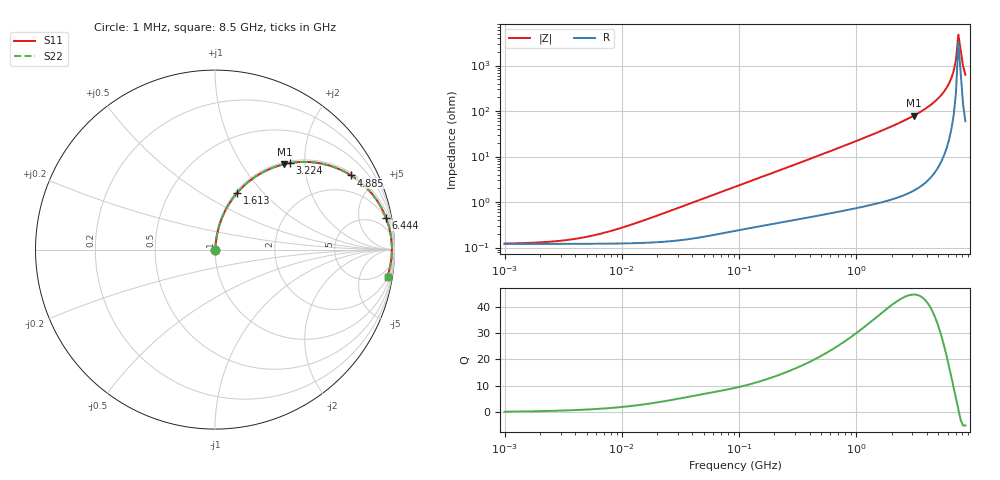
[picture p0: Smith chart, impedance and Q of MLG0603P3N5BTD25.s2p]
! S-Parameter Data Generated by TDK Corporation
! Copyright(C) 2025 TDK Corporation.
! All Rights Reserved.
! TDK P/N: MLG0603P3N5BTD25 (SMD / SMT Inductor (Coil))
! Property: L=3.5nH at 500MHz
! Size(LxWxT): 0.6x0.3x0.3mm
! Model Type: s2p (Touchstone File Format Version 1.0)
! Frequency: DC=Yes Start=1MHz Stop=8500MHz 198points Log-sweep
! Model Generated on Feb. 6, 2025
! Terms and conditions regarding TDK Simulation Models:
! 1)This simulation model is being provided solely for informational
!  purposes. Please refer to the specifications of the products in
!  terms of detailed characteristics of such products.
! 2)In no event shall TDK Corporation of any of its subsidiaries be
!  liable for any loss or damage arising, directly or indirectly,
!  from any information contained in this simulation model, including,
!  but not limited to loss or damages arising from any inaccuracies,
!  omissions or errors in connection with such information.
! 3)Any and all copyrights on this simulation model are owned by
!  TDK Corporation.  Duplication or redistribution of this simulation
!  model without prior written permission from TDK Corporation
!  is prohibited.
! 4)This simulation model is subject to any modification or change
!  without any prior notice.
! 5)Neither TDK Corporation nor any of its subsidiaries shall make any
!  warranty, express or implied, including but not limited to the
!  correctness, implied warranties of merchantability and fitness for
!  a particular purpose with respect to this simulation models.
! 6)The use of this simulation model shall be deemed to have consented
!  to the terms and conditions hereof.
! Port Assignments:
!  1 ---@@@--- 2
! Applicable Conditions:
!  Temperature = 25 degC
!  DC Bias Current = 0 A
!  Small Signal Operation
# Hz S MA R 50
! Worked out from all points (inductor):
!   197 points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, 1 MHz to 8.5 GHz, reference 50 ohm
!   read as one part in series: L = 3.87 nH near 15.95 MHz
!   highest Q = 44.5 at 3.079 GHz (marker M1), where L = 4.09 nH
!   self-resonance near 7.401 GHz
!   S11 on the Smith chart (normalised r, x): 1 MHz: 1.00, +0.00; 1.613 GHz: 1.02, +0.73; 3.224 GHz: 1.04, +1.69; 4.885 GHz: 1.11, +3.62; 6.444 GHz: 2, +10; 8.5 GHz: 2, -12
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1000000  0.001223 11.5  0.9988 -0.0  0.9988 -0.0  0.001223 11.5
2403882  0.001336 26.0  0.9988 -0.0  0.9988 -0.0  0.001336 26.0
4587603  0.001644 42.8  0.9988 -0.1  0.9988 -0.1  0.001644 42.8
8755050  0.002458 60.1  0.9988 -0.1  0.9988 -0.1  0.002458 60.1
2.10461e7  0.00527 75.2  0.9987 -0.3  0.9987 -0.3  0.00527 75.2
9.219544e7  0.02144 82.6  0.9975 -1.2  0.9975 -1.2  0.02144 82.6
4.229561e8  0.09254 81.8  0.991 -5.3  0.991 -5.3  0.09254 81.8
9.270694e8  0.1984 76.6  0.9733 -11.4  0.9733 -11.4  0.1984 76.6
1.613203e9  0.3386 68.7  0.9319 -19.8  0.9319 -19.8  0.3386 68.7
1.940355e9  0.4035 64.8  0.905 -23.8  0.905 -23.8  0.4035 64.8
3.07866e9  0.6136 50.9  0.776 -37.8  0.776 -37.8  0.6136 50.9
3.224109e9  0.6381 49.1  0.7557 -39.6  0.7557 -39.6  0.6381 49.1
4.061159e9  0.7657 38.7  0.6249 -50.0  0.6249 -50.0  0.7657 38.7
4.884749e9  0.8644 28.5  0.478 -59.8  0.478 -59.8  0.8644 28.5
5.610304e9  0.9265 19.9  0.341 -67.8  0.341 -67.8  0.9265 19.9
6.152938e9  0.9576 13.8  0.2384 -73.0  0.2384 -73.0  0.9576 13.8
6.44363e9  0.9693 10.6  0.1844 -75.2  0.1844 -75.2  0.9693 10.6
6.748056e9  0.978 7.4  0.1291 -76.5  0.1291 -76.5  0.978 7.4
7.066863e9  0.9836 4.1  0.07321 -75.0  0.07321 -75.0  0.9836 4.1
7.400733e9  0.9858 0.9  0.02043 -45.7  0.02043 -45.7  0.9858 0.9
8.116539e9  0.9805 -5.7  0.1002 75.9  0.1002 75.9  0.9805 -5.7
8.5e9  0.973 -8.9  0.1559 75.6  0.1559 75.6  0.973 -8.9
